|   IBIS model for TI xxx DSP
[IBIS Ver]   5.1
[Disclaimer]   Please be aware that in the absence of a written agreement
|   Texas Instruments(TI) assumes no liability for:
|   (1) The accuracy of the IBIS models provided to your company,
|   however, the IBIS model is compliant to industry standard
|   IQ Level 2a.  Refer to IBIS Quality Section below for
|   for full details.
|   (2) The proper functioning of these Models in your design
|   or for any resulting applications
|   (3) Infringement of patents, copyrights or intellectual
|   property rights resulting from your use of these
|   models.
|   TI provides IBIS Models as a service to our customers and
|   therefore reserves the right to limit distribution of the
|   Models.  The information is subject to change without notice.
[File Name]  j721s2_v0p3.ibs
[File Rev]   0.3
|   -Corrected differential pin mapping
[Date]   21Jun 2022
[Source]   Texas Instruments Incorporated
[Copyright]   Property of Texas Instruments Incorporated.
|   Unauthorized reproduction and/or distribution is strictly.
|   prohibited.
|   This product is protected under copyright law and trade
|   secret law as an unpublished work.
|   Created 2012,(C) Copyright 1999-2012,
|   Texas Instruments Incorporated., All Rights Reserved.
|   These commodities are under the U.S. Government
|   distribution license control. As such,they are not to be
|   re-exported without the prior approval of the U.S.
|   Department of Commerce.
[Notes]
   This file does not include AMI models for the following:
   1. PCIe
   2. CSI
   3. Display Port
   4. USB2
   5. USB3
   6. MPHY
   For SerDes simulations use Texas Instruments IBIS AMI models
   Some IV curves contain Non monotonic data points.
|   Revision History
|   GERNERAL COMMENT: All IBIS Quality Notes below reflect latest release
|   and version of IBIS File
|   File passes ibischk6.0 with 0 errors and 95 warnings
|   v0.1: Initial version
|   v0.2: Removed 4X models
|   v0.3: Corrected differential pin mapping
|   Component j721s2
[Component] j721s2
[Manufacturer] Texas Instruments
[Package]
|Variable   Typ   Min   Max
R_pkg   0.50566   0.040052   0.94543
L_pkg   3.105e-9   5.481e-10   5.565e-9
C_pkg   1.485e-12   4.706e-13   2.385e-12
[Package Model]   ibis_package_061021
[Pin]  Signal_name   model_name
H25	ATEST0   NC
L26	ATEST1   NC
T21	CAP_VDDS0	POWER
J20	CAP_VDDS0_MCU	POWER
G16	CAP_VDDS1_MCU	POWER
P21	CAP_VDDS2	POWER
H17	CAP_VDDS2_MCU	POWER
M22	CAP_VDDS5	POWER
AC20	CSI0_ATB_0_H	NC
AC19	CSI0_ATB_1_H	NC
AH19	CSI0_RXCLKN	NC
AH20	CSI0_RXCLKP	NC
AG18	CSI0_RXN0	NC
AF19	CSI0_RXN1	NC
AE18	CSI0_RXN2	NC
AD19	CSI0_RXN3	NC
AG19	CSI0_RXP0	NC
AF20	CSI0_RXP1	NC
AE19	CSI0_RXP2	NC
AD20	CSI0_RXP3	NC
AC18	CSI0_RXRCALIB	NC
AC23	CSI1_ATB_0_H	NC
AB22	CSI1_ATB_1_H	NC
AH22	CSI1_RXCLKN	NC
AH23	CSI1_RXCLKP	NC
AG21	CSI1_RXN0	NC
AF22	CSI1_RXN1	NC
AE21	CSI1_RXN2	NC
AD22	CSI1_RXN3	NC
AG22	CSI1_RXP0	NC
AF23	CSI1_RXP1	NC
AE22	CSI1_RXP2	NC
AD23	CSI1_RXP3	NC
AC21	CSI1_RXRCALIB	NC
T7	DDR0_ATB0	NC
N8	DDR0_ATB1	NC
P3	DDR0_CA0	DDR_SE
P5	DDR0_CA1	DDR_SE
N5	DDR0_CA2	DDR_SE
P2	DDR0_CA3	DDR_SE
P4	DDR0_CA4	DDR_SE
R3	DDR0_CA5	DDR_SE
R8	DDR0_CAL0	DDR_SE
R2	DDR0_CKE0	DDR_SE
R4	DDR0_CKE1	DDR_SE
R1	DDR0_CKN	DDR_DIFF
P1	DDR0_CKP	DDR_DIFF
V5	DDR0_CSN0_0	DDR_SE
W5	DDR0_CSN0_1	DDR_SE
T5	DDR0_CSN1_0	DDR_SE
U6	DDR0_CSN1_1	DDR_SE
H5	DDR0_DM0	DDR_SE
M3	DDR0_DM1	DDR_SE
U4	DDR0_DM2	DDR_SE
AD1	DDR0_DM3	DDR_SE
F3	DDR0_DQ0	DDR_SE
G4	DDR0_DQ1	DDR_SE
K3	DDR0_DQ10	DDR_SE
K1	DDR0_DQ11	DDR_SE
N4	DDR0_DQ12	DDR_SE
N2	DDR0_DQ13	DDR_SE
L4	DDR0_DQ14	DDR_SE
L2	DDR0_DQ15	DDR_SE
T1	DDR0_DQ16	DDR_SE
T3	DDR0_DQ17	DDR_SE
V3	DDR0_DQ18	DDR_SE
U2	DDR0_DQ19	DDR_SE
F5	DDR0_DQ2	DDR_SE
W2	DDR0_DQ20	DDR_SE
W4	DDR0_DQ21	DDR_SE
Y1	DDR0_DQ22	DDR_SE
Y3	DDR0_DQ23	DDR_SE
AB3	DDR0_DQ24	DDR_SE
AA2	DDR0_DQ25	DDR_SE
AA4	DDR0_DQ26	DDR_SE
Y5	DDR0_DQ27	DDR_SE
AC2	DDR0_DQ28	DDR_SE
AB5	DDR0_DQ29	DDR_SE
F1	DDR0_DQ3	DDR_SE
AD2	DDR0_DQ30	DDR_SE
AC4	DDR0_DQ31	DDR_SE
J4	DDR0_DQ4	DDR_SE
H3	DDR0_DQ5	DDR_SE
J2	DDR0_DQ6	DDR_SE
G2	DDR0_DQ7	DDR_SE
K5	DDR0_DQ8	DDR_SE
M5	DDR0_DQ9	DDR_SE
H1	DDR0_DQS0N	DDR_DIFF
G1	DDR0_DQS0P	DDR_DIFF
M1	DDR0_DQS1N	DDR_DIFF
L1	DDR0_DQS1P	DDR_DIFF
U1	DDR0_DQS2N	DDR_DIFF
V1	DDR0_DQS2P	DDR_DIFF
AC1	DDR0_DQS3N	DDR_DIFF
AB1	DDR0_DQS3P	DDR_DIFF
R5	DDR0_RESETN	DDR_SE
T8	DDR0_RET	DDR_SE
F13	DDR1_ATB0	NC
G11	DDR1_ATB1	NC
C10	DDR1_CA0	DDR_SE
E10	DDR1_CA1	DDR_SE
E9	DDR1_CA2	DDR_SE
B10	DDR1_CA3	DDR_SE
D10	DDR1_CA4	DDR_SE
C9	DDR1_CA5	DDR_SE
E8	DDR1_CAL0	DDR_SE
B9	DDR1_CKE0	DDR_SE
D9	DDR1_CKE1	DDR_SE
A9	DDR1_CKN	DDR_DIFF
A10	DDR1_CKP	DDR_DIFF
F9	DDR1_CSN0_0	DDR_SE
F8	DDR1_CSN0_1	DDR_SE
F11	DDR1_CSN1_0	DDR_SE
F10	DDR1_CSN1_1	DDR_SE
D16	DDR1_DM0	DDR_SE
E13	DDR1_DM1	DDR_SE
F7	DDR1_DM2	DDR_SE
B3	DDR1_DM3	DDR_SE
B18	DDR1_DQ0	DDR_SE
E17	DDR1_DQ1	DDR_SE
C13	DDR1_DQ10	DDR_SE
C11	DDR1_DQ11	DDR_SE
E11	DDR1_DQ12	DDR_SE
A11	DDR1_DQ13	DDR_SE
B12	DDR1_DQ14	DDR_SE
D12	DDR1_DQ15	DDR_SE
B7	DDR1_DQ16	DDR_SE
D7	DDR1_DQ17	DDR_SE
C8	DDR1_DQ18	DDR_SE
A8	DDR1_DQ19	DDR_SE
D18	DDR1_DQ2	DDR_SE
C6	DDR1_DQ20	DDR_SE
E6	DDR1_DQ21	DDR_SE
B5	DDR1_DQ22	DDR_SE
D5	DDR1_DQ23	DDR_SE
B1	DDR1_DQ24	DDR_SE
A4	DDR1_DQ25	DDR_SE
C4	DDR1_DQ26	DDR_SE
E4	DDR1_DQ27	DDR_SE
D1	DDR1_DQ28	DDR_SE
D3	DDR1_DQ29	DDR_SE
A17	DDR1_DQ3	DDR_SE
C2	DDR1_DQ30	DDR_SE
E2	DDR1_DQ31	DDR_SE
E15	DDR1_DQ4	DDR_SE
B16	DDR1_DQ5	DDR_SE
C15	DDR1_DQ6	DDR_SE
C17	DDR1_DQ7	DDR_SE
B14	DDR1_DQ8	DDR_SE
D14	DDR1_DQ9	DDR_SE
A15	DDR1_DQS0N	DDR_DIFF
A16	DDR1_DQS0P	DDR_DIFF
A12	DDR1_DQS1N	DDR_DIFF
A13	DDR1_DQS1P	DDR_DIFF
A7	DDR1_DQS2N	DDR_DIFF
A6	DDR1_DQS2P	DDR_DIFF
A2	DDR1_DQS3N	DDR_DIFF
A3	DDR1_DQS3P	DDR_DIFF
F12	DDR1_RESETN	DDR_SE
J10	DDR1_RET	DDR_SE
AE11	DP0_AUX_ATB_0	NC
AD12	DP0_AUX_ATB_1	NC
AG11	DP0_AUXN	NC
AF11	DP0_AUXP	NC
AC12	DSI0_ATB_0_H	NC
AC14	DSI0_ATB_1_H	NC
AH13	DSI0_TXCLKN	NC
AH14	DSI0_TXCLKP	NC
AG12	DSI0_TXN0	NC
AF13	DSI0_TXN1	NC
AE12	DSI0_TXN2	NC
AD13	DSI0_TXN3	NC
AG13	DSI0_TXP0	NC
AF14	DSI0_TXP1	NC
AE13	DSI0_TXP2	NC
AD14	DSI0_TXP3	NC
AC13	DSI0_TXRCALIB	NC
AC17	DSI1_ATB_0_H	NC
AC16	DSI1_ATB_1_H	NC
AH16	DSI1_TXCLKN	NC
AH17	DSI1_TXCLKP	NC
AG15	DSI1_TXN0	NC
AF16	DSI1_TXN1	NC
AE15	DSI1_TXN2	NC
AD16	DSI1_TXN3	NC
AG16	DSI1_TXP0	NC
AF17	DSI1_TXP1	NC
AE16	DSI1_TXP2	NC
AD17	DSI1_TXP3	NC
AC15	DSI1_TXRCALIB	NC
AB26	ECAP0_IN_APWM_OUT	LVCMOS_H
A27	EMU0	LVCMOS_V
C26	EMU1	LVCMOS_V
AD28	EXT_REFCLK1	LVCMOS_H
AG24	EXTINTN	IIC_H
V23	GPIO0_11	LVCMOS_H
T26	GPIO0_12	LVCMOS_H
AH25	I2C0_SCL	IIC_H
AE24	I2C0_SDA	IIC_H
N28	IFORCE	NC
L23	MAIN_ATEST	NC
U28	MCAN0_RX	LVCMOS_H
W28	MCAN0_TX	LVCMOS_H
R27	MCAN1_RX	LVCMOS_H
V26	MCAN1_TX	LVCMOS_H
AC24	MCAN12_RX	LVCMOS_H
W25	MCAN12_TX	LVCMOS_H
AF28	MCAN13_RX	LVCMOS_H
AE28	MCAN13_TX	LVCMOS_H
W23	MCAN14_RX	LVCMOS_H
AD25	MCAN14_TX	LVCMOS_H
AA23	MCAN15_RX	LVCMOS_H
Y24	MCAN15_TX	LVCMOS_H
AB24	MCAN16_RX	LVCMOS_H
Y28	MCAN16_TX	LVCMOS_H
Y25	MCAN2_RX	LVCMOS_H
R28	MCAN2_TX	LVCMOS_H
AB28	MCASP0_ACLKX	LVCMOS_H
U27	MCASP0_AFSX	LVCMOS_H
AC28	MCASP0_AXR0	LVCMOS_H
Y26	MCASP0_AXR1	LVCMOS_H
V25	MCASP0_AXR10	LVCMOS_H
T24	MCASP0_AXR11	LVCMOS_H
AB25	MCASP0_AXR12	LVCMOS_H
T23	MCASP0_AXR13	LVCMOS_H
U24	MCASP0_AXR14	LVCMOS_H
AC25	MCASP0_AXR15	LVCMOS_H
AB27	MCASP0_AXR2	LVCMOS_H
T27	MCASP0_AXR3	LVCMOS_H
U26	MCASP0_AXR4	LVCMOS_H
AA28	MCASP0_AXR5	LVCMOS_H
AD27	MCASP0_AXR6	LVCMOS_H
T25	MCASP0_AXR7	LVCMOS_H
W24	MCASP0_AXR8	LVCMOS_H
AA25	MCASP0_AXR9	LVCMOS_H
AA24	MCASP1_ACLKX	LVCMOS_H
V28	MCASP1_AFSX	LVCMOS_H
T28	MCASP1_AXR0	LVCMOS_H
V27	MCASP1_AXR1	LVCMOS_H
W27	MCASP1_AXR2	LVCMOS_H
AD26	MCASP1_AXR3	LVCMOS_H
U25	MCASP1_AXR4	LVCMOS_H
Y27	MCASP2_ACLKX	LVCMOS_H
AA27	MCASP2_AFSX	LVCMOS_H
AA26	MCASP2_AXR0	LVCMOS_H
AC27	MCASP2_AXR1	LVCMOS_H
L25	MCU_ADC0_AIN0	NC
K25	MCU_ADC0_AIN1	NC
M24	MCU_ADC0_AIN2	NC
L24	MCU_ADC0_AIN3	NC
L27	MCU_ADC0_AIN4	NC
K24	MCU_ADC0_AIN5	NC
M27	MCU_ADC0_AIN6	NC
M26	MCU_ADC0_AIN7	NC
P25	MCU_ADC1_AIN0	NC
R25	MCU_ADC1_AIN1	NC
P28	MCU_ADC1_AIN2	NC
P27	MCU_ADC1_AIN3	NC
N25	MCU_ADC1_AIN4	NC
P26	MCU_ADC1_AIN5	NC
N26	MCU_ADC1_AIN6	NC
N27	MCU_ADC1_AIN7	NC
G24	MCU_I2C0_SCL	IIC_V
J25	MCU_I2C0_SDA	IIC_V
E28	MCU_MCAN0_RX	LVCMOS_V
E27	MCU_MCAN0_TX	LVCMOS_V
A21	MCU_MDIO0_MDC	LVCMOS_V
A22	MCU_MDIO0_MDIO	LVCMOS_V
D19	MCU_OSPI0_CLK	LVCMOS_V
F15	MCU_OSPI0_CSN0	LVCMOS_V
G17	MCU_OSPI0_CSN1	LVCMOS_V
F14	MCU_OSPI0_CSN2	LVCMOS_V
F17	MCU_OSPI0_CSN3	LVCMOS_V
C19	MCU_OSPI0_D0	LVCMOS_V
F16	MCU_OSPI0_D1	LVCMOS_V
G15	MCU_OSPI0_D2	LVCMOS_V
F18	MCU_OSPI0_D3	LVCMOS_V
E19	MCU_OSPI0_D4	LVCMOS_V
G19	MCU_OSPI0_D5	LVCMOS_V
F19	MCU_OSPI0_D6	LVCMOS_V
F20	MCU_OSPI0_D7	LVCMOS_V
E18	MCU_OSPI0_DQS	LVCMOS_V
E20	MCU_OSPI0_LBCLKO	LVCMOS_V
A19	MCU_OSPI1_CLK	LVCMOS_V
D20	MCU_OSPI1_CSN0	LVCMOS_V
C21	MCU_OSPI1_CSN1	LVCMOS_V
D21	MCU_OSPI1_D0	LVCMOS_V
G20	MCU_OSPI1_D1	LVCMOS_V
C20	MCU_OSPI1_D2	LVCMOS_V
A20	MCU_OSPI1_D3	LVCMOS_V
B19	MCU_OSPI1_DQS	LVCMOS_V
B20	MCU_OSPI1_LBCLKO	LVCMOS_V
G23	MCU_PORZ	RESET_H
A23	MCU_RESETSTATZ	LVCMOS_V
A26	MCU_RESETZ	LVCMOS_V
B22	MCU_RGMII1_RD0	LVCMOS_V
B21	MCU_RGMII1_RD1	LVCMOS_V
C22	MCU_RGMII1_RD2	LVCMOS_V
D23	MCU_RGMII1_RD3	LVCMOS_V
E23	MCU_RGMII1_RX_CTL	LVCMOS_V
D22	MCU_RGMII1_RXC	LVCMOS_V
F23	MCU_RGMII1_TD0	LVCMOS_V
G22	MCU_RGMII1_TD1	LVCMOS_V
E21	MCU_RGMII1_TD2	LVCMOS_V
E22	MCU_RGMII1_TD3	LVCMOS_V
F22	MCU_RGMII1_TX_CTL	LVCMOS_V
F21	MCU_RGMII1_TXC	LVCMOS_V
J23	MCU_SAFETY_ERRORN	LVCMOS_V
B27	MCU_SPI0_CLK	LVCMOS_V
B26	MCU_SPI0_CS0	LVCMOS_V
D24	MCU_SPI0_D0	LVCMOS_V
B25	MCU_SPI0_D1	LVCMOS_V
AF1	MMC0_CALPAD	EMMC
AC6	MMC0_CLK	EMMC
AF2	MMC0_CMD	EMMC
AF4	MMC0_DAT0	EMMC
AD3	MMC0_DAT1	EMMC
AD4	MMC0_DAT2	EMMC
AF3	MMC0_DAT3	EMMC
AE2	MMC0_DAT4	EMMC
AG3	MMC0_DAT5	EMMC
AE1	MMC0_DAT6	EMMC
AG1	MMC0_DAT7	EMMC
AE3	MMC0_DS	EMMC
AD5	MMC0_VCTRL_TP	EMMC
P23	MMC1_CLK	SDIO_H
N24	MMC1_CMD	SDIO_H
M23	MMC1_DAT0	SDIO_H
P24	MMC1_DAT1	SDIO_H
R24	MMC1_DAT2	SDIO_H
R22	MMC1_DAT3	SDIO_H
M28	OSC1_XI	NC
L28	OSC1_XO	NC
AH10	PCIE_REFCLK1_N_OUT	NC
AH11	PCIE_REFCLK1_P_OUT	NC
G26	PMIC_POWER_EN1	LVCMOS_V
AD24	PMIC_WAKE0	LVCMOS_H
K23	PORZ	RESET_H
A24	RESET_REQZ	LVCMOS_V
AF27	RESETSTATZ	LVCMOS_H
AD11	SERDES0_ATB_0	NC
AD10	SERDES0_ATB_1	NC
AH4	SERDES0_REFCLK_N	NC
AH5	SERDES0_REFCLK_P	NC
AC10	SERDES0_REXT	NC
AF9	SERDES0_RX0_N	NC
AF10	SERDES0_RX0_P	NC
AE8	SERDES0_RX1_N	NC
AE9	SERDES0_RX1_P	NC
AF6	SERDES0_RX2_N	NC
AF7	SERDES0_RX2_P	NC
AE5	SERDES0_RX3_N	NC
AE6	SERDES0_RX3_P	NC
AH7	SERDES0_TX0_N	NC
AH8	SERDES0_TX0_P	NC
AG8	SERDES0_TX1_N	NC
AG9	SERDES0_TX1_P	NC
AG5	SERDES0_TX2_N	NC
AG6	SERDES0_TX2_P	NC
AD7	SERDES0_TX3_N	NC
AD8	SERDES0_TX3_P	NC
AF25	SOC_SAFETY_ERRORN	LVCMOS_H
AH27	SPI0_CLK	LVCMOS_H
AE27	SPI0_CS0	LVCMOS_H
AF26	SPI0_CS1	LVCMOS_H
AG26	SPI0_D0	LVCMOS_H
AH26	SPI0_D1	LVCMOS_H
A25	TCK	LVCMOS_V
AG28	TDI	LVCMOS_H
AE26	TDO	LVCMOS_H
G21	TEMP_DIODE_P	NC
AE25	TIMER_IO0	LVCMOS_H
AG25	TIMER_IO1	LVCMOS_H
AG27	TMS	LVCMOS_H
B28	TRSTN	LVCMOS_V
AG2	USB0_DM	NC
AH2	USB0_DP	NC
AC9	USB0_ID	NC
AA6	USB0_RCALIB	NC
AA8	USB0_VBUS	NC
J13	VDD_CORE	POWER
J15	VDD_CORE	POWER
M16	VDD_CORE	POWER
M19	VDD_CORE	POWER
N10	VDD_CORE	POWER
P18	VDD_CORE	POWER
R17	VDD_CORE	POWER
R19	VDD_CORE	POWER
T10	VDD_CORE	POWER
T20	VDD_CORE	POWER
U8	VDD_CORE	POWER
U15	VDD_CORE	POWER
U17	VDD_CORE	POWER
V7	VDD_CORE	POWER
V9	VDD_CORE	POWER
V14	VDD_CORE	POWER
V18	VDD_CORE	POWER
V20	VDD_CORE	POWER
W8	VDD_CORE	POWER
W10	VDD_CORE	POWER
W13	VDD_CORE	POWER
W15	VDD_CORE	POWER
W17	VDD_CORE	POWER
W19	VDD_CORE	POWER
W21	VDD_CORE	POWER
Y9	VDD_CORE	POWER
Y12	VDD_CORE	POWER
Y22	VDD_CORE	POWER
AA21	VDD_CORE	POWER
AB20	VDD_CORE	POWER
G8	VDD_CPU	POWER
H7	VDD_CPU	POWER
J8	VDD_CPU	POWER
K7	VDD_CPU	POWER
K9	VDD_CPU	POWER
K11	VDD_CPU	POWER
K13	VDD_CPU	POWER
L8	VDD_CPU	POWER
M7	VDD_CPU	POWER
M9	VDD_CPU	POWER
M14	VDD_CPU	POWER
N11	VDD_CPU	POWER
N15	VDD_CPU	POWER
P16	VDD_CPU	POWER
R13	VDD_CPU	POWER
R15	VDD_CPU	POWER
T12	VDD_CPU	POWER
T14	VDD_CPU	POWER
U11	VDD_CPU	POWER
U13	VDD_CPU	POWER
K16	VDD_MCU	POWER
K18	VDD_MCU	POWER
L15	VDD_MCU	POWER
L17	VDD_MCU	POWER
L19	VDD_MCU	POWER
J19	VDD_MCU_WAKE1	POWER
P20	VDD_WAKE0	POWER
AB17	VDDA_0P8_CSIRX0_1	POWER
AB18	VDDA_0P8_CSIRX0_1	POWER
W7	VDDA_0P8_DLL_MMC0	POWER
AB14	VDDA_0P8_DSITX	POWER
AB15	VDDA_0P8_DSITX_C	POWER
P10	VDDA_0P8_PLL_DDR0	POWER
J14	VDDA_0P8_PLL_DDR1	POWER
AA10	VDDA_0P8_SERDES_C0_1	POWER
AA11	VDDA_0P8_SERDES_C0_1	POWER
AB10	VDDA_0P8_SERDES0_1	POWER
AB11	VDDA_0P8_SERDES0_1	POWER
AB8	VDDA_0P8_USB	POWER
AA17	VDDA_1P8_CSIRX0_1	POWER
AA19	VDDA_1P8_CSIRX0_1	POWER
AA14	VDDA_1P8_DSITX	POWER
AA15	VDDA_1P8_DSITX	POWER
AA12	VDDA_1P8_SERDES0_1	POWER
AB13	VDDA_1P8_SERDES2_4	POWER
AB7	VDDA_1P8_USB	POWER
AB9	VDDA_3P3_USB	POWER
J21	VDDA_ADC0	POWER
K21	VDDA_ADC1	POWER
K22	VDDA_MCU_PLLGRP0	POWER
J17	VDDA_MCU_TEMP	POWER
L21	VDDA_OSC1	POWER
U18	VDDA_PLLGRP0	POWER
V19	VDDA_PLLGRP1	POWER
Y16	VDDA_PLLGRP10	POWER
Y18	VDDA_PLLGRP12	POWER
V12	VDDA_PLLGRP13	POWER
Y11	VDDA_PLLGRP2	POWER
N14	VDDA_PLLGRP5	POWER
R12	VDDA_PLLGRP6	POWER
R11	VDDA_PLLGRP7	POWER
K12	VDDA_PLLGRP8	POWER
T18	VDDA_PLLGRP9	POWER
L20	VDDA_POR_WKUP	POWER
U19	VDDA_TEMP0	POWER
K10	VDDA_TEMP1	POWER
T16	VDDA_TEMP2	POWER
U10	VDDA_TEMP3	POWER
Y14	VDDA_TEMP4	POWER
J22	VDDA_WKUP	POWER
N17	VDDAR_CORE	POWER
V11	VDDAR_CORE	POWER
V16	VDDAR_CORE	POWER
Y20	VDDAR_CORE	POWER
H9	VDDAR_CPU	POWER
K14	VDDAR_CPU	POWER
P11	VDDAR_CPU	POWER
P14	VDDAR_CPU	POWER
V13	VDDAR_CPU	POWER
K17	VDDAR_MCU	POWER
K19	VDDAR_MCU	POWER
A1	VDDS_DDR	POWER
A18	VDDS_DDR	POWER
G6	VDDS_DDR	POWER
G10	VDDS_DDR	POWER
G12	VDDS_DDR	POWER
G14	VDDS_DDR	POWER
H11	VDDS_DDR	POWER
H13	VDDS_DDR	POWER
H15	VDDS_DDR	POWER
J6	VDDS_DDR	POWER
L6	VDDS_DDR	POWER
N6	VDDS_DDR	POWER
N9	VDDS_DDR	POWER
P7	VDDS_DDR	POWER
P8	VDDS_DDR	POWER
R6	VDDS_DDR	POWER
U9	VDDS_DDR	POWER
AA1	VDDS_DDR	POWER
R9	VDDS_DDR_C0	POWER
J12	VDDS_DDR_C1	POWER
Y7	VDDS_MMC0	POWER
Y8	VDDS_MMC0	POWER
R21	VDDSHV0	POWER
U21	VDDSHV0	POWER
U22	VDDSHV0	POWER
H19	VDDSHV0_MCU	POWER
H20	VDDSHV0_MCU	POWER
H16	VDDSHV1_MCU	POWER
J16	VDDSHV1_MCU	POWER
M20	VDDSHV2	POWER
R20	VDDSHV2	POWER
G18	VDDSHV2_MCU	POWER
H18	VDDSHV2_MCU	POWER
M21	VDDSHV5	POWER
N22	VDDSHV5	POWER
H23	VMON1_ER_VSYS	POWER
M18	VMON2_IR_VCPU	POWER
L22	VMON3_IR_VEXT1P8	POWER
N19	VMON4_IR_VEXT1P8	POWER
N20	VMON5_IR_VEXT3P3	POWER
L18	VMON6_IR_VEXT1P8	POWER
V22	VPP_CORE	POWER
H22	VPP_MCU	POWER
K28	VSENSE	POWER
A5	VSS	GND
A14	VSS	GND
B2	VSS	GND
B4	VSS	GND
B6	VSS	GND
B8	VSS	GND
B11	VSS	GND
B13	VSS	GND
B15	VSS	GND
B17	VSS	GND
B23	VSS	GND
C1	VSS	GND
C3	VSS	GND
C5	VSS	GND
C7	VSS	GND
C12	VSS	GND
C14	VSS	GND
C16	VSS	GND
C18	VSS	GND
D2	VSS	GND
D4	VSS	GND
D6	VSS	GND
D8	VSS	GND
D11	VSS	GND
D13	VSS	GND
D15	VSS	GND
D17	VSS	GND
E1	VSS	GND
E3	VSS	GND
E5	VSS	GND
E7	VSS	GND
E12	VSS	GND
E14	VSS	GND
E16	VSS	GND
E26	VSS	GND
F2	VSS	GND
F4	VSS	GND
F6	VSS	GND
G3	VSS	GND
G5	VSS	GND
G7	VSS	GND
G9	VSS	GND
G13	VSS	GND
G28	VSS	GND
H2	VSS	GND
H4	VSS	GND
H6	VSS	GND
H8	VSS	GND
H10	VSS	GND
H12	VSS	GND
H14	VSS	GND
H21	VSS	GND
J1	VSS	GND
J3	VSS	GND
J5	VSS	GND
J7	VSS	GND
J9	VSS	GND
J11	VSS	GND
J18	VSS	GND
J24	VSS	GND
K2	VSS	GND
K4	VSS	GND
K6	VSS	GND
K8	VSS	GND
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|********************  DIFF PIN  *******************************
[Diff_pin]   inv_pin vdiff tdelay_typ   tdelay_min  tdelay_max
H1	G1	NA NA NA NA	||	ddr0_dqs0n	&	ddr0_dqs0p
M1	L1	NA NA NA NA	||	ddr0_dqs1n	&	ddr0_dqs1p
U1	V1	NA NA NA NA	||	ddr0_dqs2n	&	ddr0_dqs2p
AC1	AB1	NA NA NA NA	||	ddr0_dqs3n	&	ddr0_dqs3p
R1   P1	NA NA NA NA	||	ddr0_ckn	&	ddr0_ckp
A15	A16	NA NA NA NA	||	ddr1_dqs0n	&	ddr1_dqs0p
A12	A13	NA NA NA NA	||	ddr1_dqs1n	&	ddr1_dqs1p
A7	A6	NA NA NA NA	||	ddr1_dqs2n	&	ddr1_dqs2p
A2	A3	NA NA NA NA	||	ddr1_dqs3n	&	ddr1_dqs3p
A9	A10	NA NA NA NA	||	ddr1_ckn	&	ddr1_ckp
[Series Pin Mapping] pin_2 model_name function_table_group
| AC25	AD25	s_ILVDS18TH_PB300
| AD24	AE24	s_ILVDS18TH_PB300
| K21	L21	s_ILVDS18TH_PB300
|---------------- DDR -------------------
[Model Selector] DDR_SE
lpddr4_ocd_240p_240n  driver with 240 ohms pullup and 240 ohms pulldown strength
lpddr4_ocd_120p_120n  driver with 120 ohms pullup and 120 ohms pulldown strength
lpddr4_ocd_80p_80n  driver with 80 ohms pullup and 80 ohms pulldown strength
lpddr4_ocd_60p_60n  driver with 60 ohms pullup and 60 ohms pulldown strength
lpddr4_ocd_48p_48n  driver with 48 ohms pullup and 48 ohms pulldown strength
lpddr4_ocd_40p_40n  driver with 40 ohms pullup and 40 ohms pulldown strength
lpddr4_ocd_120pd_60p_40n  driver with 60/40 ohms pullup/pulldown 120 ohms aopd strength
lpddr4_ocd_120pd_48p_40n  driver with 48/40 ohms pullup/pulldown 120 ohms aopd strength
lpddr4_odt_240  240 ohm termination
lpddr4_odt_120  120 ohm termination
lpddr4_odt_80  80 ohm termination
lpddr4_odt_60  60 ohm termination
lpddr4_odt_48  48 ohm termination
lpddr4_odt_40  40 ohm termination
lpddr4_odt_off  open ohm termination
[Model Selector] DDR_DIFF
lpddr4_ocd_240p_240n_diff  driver with 240 ohms pullup and 240 ohms pulldown strength
lpddr4_ocd_120p_120n_diff  driver with 120 ohms pullup and 120 ohms pulldown strength
lpddr4_ocd_80p_80n_diff  driver with 80 ohms pullup and 80 ohms pulldown strength
lpddr4_ocd_60p_60n_diff  driver with 60 ohms pullup and 60 ohms pulldown strength
lpddr4_ocd_48p_48n_diff  driver with 48 ohms pullup and 48 ohms pulldown strength
lpddr4_ocd_40p_40n_diff  driver with 40 ohms pullup and 40 ohms pulldown strength
lpddr4_ocd_120pd_60p_40n_diff  driver with 60/40 ohms pullup/pulldown 120 ohms aopd strength
lpddr4_ocd_120pd_48p_40n_diff  driver with 48/40 ohms pullup/pulldown 120 ohms aopd strength
lpddr4_odt_240_diff  240 ohm termination
lpddr4_odt_120_diff  120 ohm termination
lpddr4_odt_80_diff  80 ohm termination
lpddr4_odt_60_diff  60 ohm termination
lpddr4_odt_48_diff  48 ohm termination
lpddr4_odt_40_diff  40 ohm termination
lpddr4_odt_off_diff  open ohm termination
|****************** SDIO
[Model Selector] SDIO_H
sdio1_r33_1p8_h PRWDWUWSWEWCDGSDIO_H@_R33_1p8_comment
sdio1_r33_3p3_h PRWDWUWSWEWCDGSDIO_H@_R33_3p3_comment
sdio1_r40_1p8_h PRWDWUWSWEWCDGSDIO_H@_R40_1p8_comment
sdio1_r40_3p3_h PRWDWUWSWEWCDGSDIO_H@_R40_3p3_comment
sdio1_r50_1p8_h PRWDWUWSWEWCDGSDIO_H@_R50_1p8_comment
sdio1_r50_3p3_h PRWDWUWSWEWCDGSDIO_H@_R50_3p3_comment
sdio1_r66_1p8_h PRWDWUWSWEWCDGSDIO_H@_R66_1p8_comment
sdio1_r66_3p3_h PRWDWUWSWEWCDGSDIO_H@_R66_3p3_comment
sdio1_utr33_1p8_h PRWDWUWSWEWCDGSDIO_H@_UT_R33_1p8_comment
sdio1_utr33_3p3_h PRWDWUWSWEWCDGSDIO_H@_UT_R33_3p3_comment
sdio1_utr40_1p8_h PRWDWUWSWEWCDGSDIO_H@_UT_R40_1p8_comment
sdio1_utr40_3p3_h PRWDWUWSWEWCDGSDIO_H@_UT_R40_3p3_comment
sdio1_utr50_1p8_h PRWDWUWSWEWCDGSDIO_H@_UT_R50_1p8_comment
sdio1_utr50_3p3_h PRWDWUWSWEWCDGSDIO_H@_UT_R50_3p3_comment
sdio1_utr66_1p8_h PRWDWUWSWEWCDGSDIO_H@_UT_R66_1p8_comment
sdio1_utr66_3p3_h PRWDWUWSWEWCDGSDIO_H@_UT_R66_3p3_comment
|********** LVCMOS
[Model Selector] LVCMOS_H
lvcmos1_nom_1p8_h PRWDWUWSWEWCDGLVCMOS_H@_Nom_1p8_comment
lvcmos1_nom_3p3_h PRWDWUWSWEWCDGLVCMOS_H@_Nom_3p3_comment
lvcmos1_slow_1p8_h PRWDWUWSWEWCDGLVCMOS_H@_Slow_1p8_comment
lvcmos1_slow_3p3_h PRWDWUWSWEWCDGLVCMOS_H@_Slow_3p3_comment
lvcmos1_fast_1p8_h PRWDWUWSWEWCDGLVCMOS_H@_Fast_1p8_comment
lvcmos1_fast_3p3_h PRWDWUWSWEWCDGLVCMOS_H@_Fast_3p3_comment
lvcmos1_utnom_1p8_h PRWDWUWSWEWCDGLVCMOS_H@_UT_Nom_1p8_comment
lvcmos1_utnom_3p3_h PRWDWUWSWEWCDGLVCMOS_H@_UT_Nom_3p3_comment
lvcmos1_utslow_1p8_h PRWDWUWSWEWCDGLVCMOS_H@_UT_Slow_1p8_comment
lvcmos1_utslow_3p3_h PRWDWUWSWEWCDGLVCMOS_H@_UT_Slow_3p3_comment
lvcmos1_utfast_1p8_h PRWDWUWSWEWCDGLVCMOS_H@_UT_Fast_1p8_comment
lvcmos1_utfast_3p3_h PRWDWUWSWEWCDGLVCMOS_H@_UT_Fast_3p3_comment
[Model Selector] LVCMOS_V
lvcmos0_nom_1p8_v PRWDWUWSWEWCDGLVCMOS_V@_Nom_1p8_comment
lvcmos0_nom_3p3_v PRWDWUWSWEWCDGLVCMOS_V@_Nom_3p3_comment
lvcmos0_slow_1p8_v PRWDWUWSWEWCDGLVCMOS_V@_Slow_1p8_comment
lvcmos0_slow_3p3_v PRWDWUWSWEWCDGLVCMOS_V@_Slow_3p3_comment
lvcmos0_fast_1p8_v PRWDWUWSWEWCDGLVCMOS_V@_Fast_1p8_comment
lvcmos0_fast_3p3_v PRWDWUWSWEWCDGLVCMOS_V@_Fast_3p3_comment
lvcmos0_utnom_1p8_v PRWDWUWSWEWCDGLVCMOS_V@_UT_Nom_1p8_comment
lvcmos0_utnom_3p3_v PRWDWUWSWEWCDGLVCMOS_V@_UT_Nom_3p3_comment
lvcmos0_utslow_1p8_v PRWDWUWSWEWCDGLVCMOS_V@_UT_Slow_1p8_comment
lvcmos0_utslow_3p3_v PRWDWUWSWEWCDGLVCMOS_V@_UT_Slow_3p3_comment
lvcmos0_utfast_1p8_v PRWDWUWSWEWCDGLVCMOS_V@_UT_Fast_1p8_comment
lvcmos0_utfast_3p3_v PRWDWUWSWEWCDGLVCMOS_V@_UT_Fast_3p3_comment
[Model Selector] IIC_H
Cell18_0_0_H PRBOPDDGZIIC_H@HSMODE_HSMCSE=0_0_comment 1.8V
Cell18_0_1_H PRBOPDDGZIIC_H@HSMODE_HSMCSE=0_1_comment 1.8V
Cell18_0_2_H PRBOPDDGZIIC_H@HSMODE_HSMCSE=1_0_comment 1.8V
Cell18_0_3_H PRBOPDDGZIIC_H@HSMODE_HSMCSE=1_1_comment 1.8V
Cell33_0_0_H PRBOPDDGZIIC_H@HSMODE_HSMCSE=0_0_comment
Cell33_0_1_H PRBOPDDGZIIC_H@HSMODE_HSMCSE=0_1_comment
Cell33_0_2_H PRBOPDDGZIIC_H@HSMODE_HSMCSE=1_0_comment
Cell33_0_3_H PRBOPDDGZIIC_H@HSMODE_HSMCSE=1_1_comment
[Model Selector] IIC_V
Cell18_1_0 PRBOPDDGZIIC_V@HSMODE_HSMCSE=0_0_comment  1.8V
Cell18_1_1 PRBOPDDGZIIC_V@HSMODE_HSMCSE=0_1_comment  1.8V
Cell18_1_2 PRBOPDDGZIIC_V@HSMODE_HSMCSE=1_0_comment  1.8V
Cell18_1_3 PRBOPDDGZIIC_V@HSMODE_HSMCSE=1_1_comment  1.8V
Cell33_1_0 PRBOPDDGZIIC_V@HSMODE_HSMCSE=0_0_comment
Cell33_1_1 PRBOPDDGZIIC_V@HSMODE_HSMCSE=0_1_comment
Cell33_1_2 PRBOPDDGZIIC_V@HSMODE_HSMCSE=1_0_comment
Cell33_1_3 PRBOPDDGZIIC_V@HSMODE_HSMCSE=1_1_comment
|***************** RESET ************************************************
[Model Selector] RESET_H
reset18_0_0 PDIDGZRESET_H
|   EMMC
[MODEL SELECTOR] EMMC
emmc51_io_tx33ohm   33ohm DRIVER
emmc51_io_tx40ohm   40ohm DRIVER
emmc51_io_tx50ohm   50ohm DRIVER
emmc51_io_tx66ohm   66ohm DRIVER
emmc51_io_tx100ohm  100ohm DRIVER
emmc51_io_txod   Open drain DRIVER
|******************** Package Model *************************************
[Define Package Model]   ibis_package_061021
[Manufacturer]   TI
[OEM]   TI
[Description]   472-pin Package
|[Number of Sections]   1
[Number of Pins]   472
[Pin Numbers]
|[Pin Name]  Net Number   Net Name   Net's All Pins
T21   | 1   CAP_VDDS0   T21
J20   | 2   CAP_VDDS0_MCU   J20
G16   | 3   CAP_VDDS1_MCU   G16
P21   | 4   CAP_VDDS2   P21
H17   | 5   CAP_VDDS2_MCU   H17
M22   | 6   CAP_VDDS5   M22
N17   | 7   VDDAR_CORE   N17
   |V16
   |V11
   |Y20
H9   | 8   VDDAR_CPU   H9
   |K14
   |P14
   |V13
   |P11
K17   | 9   VDDAR_MCU   K17
   |K19
AB17   | 10   VDDA_0P8_CSIRX0_1   AB17
   |AB18
W7   | 11   VDDA_0P8_DLL_MMC0   W7
AB14   | 12   VDDA_0P8_DSITX   AB14
AB15   | 13   VDDA_0P8_DSITX_C   AB15
P10   | 14   VDDA_0P8_PLL_DDR0   P10
J14   | 15   VDDA_0P8_PLL_DDR1   J14
AB10   | 16   VDDA_0P8_SERDES0_1   AB10
   |AB11
AA10   | 17   VDDA_0P8_SERDES_C0_1   AA10
   |AA11
AB8   | 18   VDDA_0P8_USB   AB8
AA17   | 19   VDDA_1P8_CSIRX0_1   AA17
   |AA19
AA14   | 20   VDDA_1P8_DSITX   AA14
   |AA15
AA12   | 21   VDDA_1P8_SERDES0_1   AA12
AB13   | 22   VDDA_1P8_SERDES2_4   AB13
AB7   | 23   VDDA_1P8_USB   AB7
AB9   | 24   VDDA_3P3_USB   AB9
J21   | 25   VDDA_ADC0   J21
K21   | 26   VDDA_ADC1   K21
K22   | 27   VDDA_MCU_PLLGRP0   K22
J17   | 28   VDDA_MCU_TEMP   J17
L21   | 29   VDDA_OSC1   L21
U18   | 30   VDDA_PLLGRP0   U18
V19   | 31   VDDA_PLLGRP1   V19
Y11   | 32   VDDA_PLLGRP2   Y11
N14   | 33   VDDA_PLLGRP5   N14
R12   | 34   VDDA_PLLGRP6   R12
R11   | 35   VDDA_PLLGRP7   R11
K12   | 36   VDDA_PLLGRP8   K12
T18   | 37   VDDA_PLLGRP9   T18
Y16   | 38   VDDA_PLLGRP10   Y16
Y18   | 39   VDDA_PLLGRP12   Y18
V12   | 40   VDDA_PLLGRP13   V12
L20   | 41   VDDA_POR_WKUP   L20
U19   | 42   VDDA_TEMP0   U19
K10   | 43   VDDA_TEMP1   K10
T16   | 44   VDDA_TEMP2   T16
U10   | 45   VDDA_TEMP3   U10
Y14   | 46   VDDA_TEMP4   Y14
J22   | 47   VDDA_WKUP   J22
R21   | 48   VDDSHV0   R21
   |U21
   |U22
H19   | 49   VDDSHV0_MCU   H19
   |H20
H16   | 50   VDDSHV1_MCU   H16
   |J16
M20   | 51   VDDSHV2   M20
   |R20
G18   | 52   VDDSHV2_MCU   G18
   |H18
M21   | 53   VDDSHV5   M21
   |N22
H15   | 54   VDDS_DDR   H15
   |G14
   |A1
   |A18
   |H13
   |G12
   |H11
   |G10
   |G6
   |J6
   |L6
   |N9
   |N6
   |P8
   |P7
   |R6
   |U9
   |AA1
R9   | 55   VDDS_DDR_C0   R9
J12   | 56   VDDS_DDR_C1   J12
Y7   | 57   VDDS_MMC0   Y7
   |Y8
M19   | 58   VDD_CORE   M19
   |U17
   |V18
   |W13
   |W19
   |W21
   |Y12
   |Y22
   |AA21
   |AB20
   |J15
   |J13
   |M16
   |P18
   |R19
   |R17
   |T20
   |U15
   |N10
   |T10
   |U8
   |V20
   |V14
   |V9
   |V7
   |W17
   |W15
   |W10
   |W8
   |Y9
K11   | 59   VDD_CPU   K11
   |K13
   |K9
   |M14
   |N11
   |R13
   |T12
   |U11
   |U13
   |N15
   |P16
   |R15
   |T14
   |H7
   |G8
   |J8
   |K7
   |L8
   |M9
   |M7
K16   | 60   VDD_MCU   K16
   |K18
   |L15
   |L17
   |L19
J19   | 61   VDD_MCU_WAKE1   J19
P20   | 62   VDD_WAKE0   P20
V22   | 63   VPP_CORE   V22
H22   | 64   VPP_MCU   H22
H25   | 65   ATEST0   H25
L26   | 66   ATEST1   L26
AC20   | 67   CSI0_ATB_0_H   AC20
AC19   | 68   CSI0_ATB_1_H   AC19
AH19   | 69   CSI0_RXCLKN   AH19
AH20   | 70   CSI0_RXCLKP   AH20
AG18   | 71   CSI0_RXN0   AG18
AF19   | 72   CSI0_RXN1   AF19
AE18   | 73   CSI0_RXN2   AE18
AD19   | 74   CSI0_RXN3   AD19
AG19   | 75   CSI0_RXP0   AG19
AF20   | 76   CSI0_RXP1   AF20
AE19   | 77   CSI0_RXP2   AE19
AD20   | 78   CSI0_RXP3   AD20
AC18   | 79   CSI0_RXRCALIB   AC18
AC23   | 80   CSI1_ATB_0_H   AC23
AB22   | 81   CSI1_ATB_1_H   AB22
AH22   | 82   CSI1_RXCLKN   AH22
AH23   | 83   CSI1_RXCLKP   AH23
AG21   | 84   CSI1_RXN0   AG21
AF22   | 85   CSI1_RXN1   AF22
AE21   | 86   CSI1_RXN2   AE21
AD22   | 87   CSI1_RXN3   AD22
AG22   | 88   CSI1_RXP0   AG22
AF23   | 89   CSI1_RXP1   AF23
AE22   | 90   CSI1_RXP2   AE22
AD23   | 91   CSI1_RXP3   AD23
AC21   | 92   CSI1_RXRCALIB   AC21
T7   | 93   DDR0_ATB0   T7
N8   | 94   DDR0_ATB1   N8
P3   | 95   DDR0_CA0   P3
P5   | 96   DDR0_CA1   P5
N5   | 97   DDR0_CA2   N5
P2   | 98   DDR0_CA3   P2
P4   | 99   DDR0_CA4   P4
R3   | 100   DDR0_CA5   R3
R8   | 101   DDR0_CAL0   R8
R2   | 102   DDR0_CKE0   R2
R4   | 103   DDR0_CKE1   R4
R1   | 104   DDR0_CKN   R1
P1   | 105   DDR0_CKP   P1
V5   | 106   DDR0_CSN0_0   V5
W5   | 107   DDR0_CSN0_1   W5
T5   | 108   DDR0_CSN1_0   T5
U6   | 109   DDR0_CSN1_1   U6
H5   | 110   DDR0_DM0   H5
M3   | 111   DDR0_DM1   M3
U4   | 112   DDR0_DM2   U4
AD1   | 113   DDR0_DM3   AD1
F3   | 114   DDR0_DQ0   F3
G4   | 115   DDR0_DQ1   G4
F5   | 116   DDR0_DQ2   F5
F1   | 117   DDR0_DQ3   F1
J4   | 118   DDR0_DQ4   J4
H3   | 119   DDR0_DQ5   H3
J2   | 120   DDR0_DQ6   J2
G2   | 121   DDR0_DQ7   G2
K5   | 122   DDR0_DQ8   K5
M5   | 123   DDR0_DQ9   M5
K3   | 124   DDR0_DQ10   K3
K1   | 125   DDR0_DQ11   K1
N4   | 126   DDR0_DQ12   N4
N2   | 127   DDR0_DQ13   N2
L4   | 128   DDR0_DQ14   L4
L2   | 129   DDR0_DQ15   L2
T1   | 130   DDR0_DQ16   T1
T3   | 131   DDR0_DQ17   T3
V3   | 132   DDR0_DQ18   V3
U2   | 133   DDR0_DQ19   U2
W2   | 134   DDR0_DQ20   W2
W4   | 135   DDR0_DQ21   W4
Y1   | 136   DDR0_DQ22   Y1
Y3   | 137   DDR0_DQ23   Y3
AB3   | 138   DDR0_DQ24   AB3
AA2   | 139   DDR0_DQ25   AA2
AA4   | 140   DDR0_DQ26   AA4
Y5   | 141   DDR0_DQ27   Y5
AC2   | 142   DDR0_DQ28   AC2
AB5   | 143   DDR0_DQ29   AB5
AD2   | 144   DDR0_DQ30   AD2
AC4   | 145   DDR0_DQ31   AC4
H1   | 146   DDR0_DQS0N   H1
G1   | 147   DDR0_DQS0P   G1
M1   | 148   DDR0_DQS1N   M1
L1   | 149   DDR0_DQS1P   L1
U1   | 150   DDR0_DQS2N   U1
V1   | 151   DDR0_DQS2P   V1
AC1   | 152   DDR0_DQS3N   AC1
AB1   | 153   DDR0_DQS3P   AB1
R5   | 154   DDR0_RESETN   R5
T8   | 155   DDR0_RET   T8
F13   | 156   DDR1_ATB0   F13
G11   | 157   DDR1_ATB1   G11
C10   | 158   DDR1_CA0   C10
E10   | 159   DDR1_CA1   E10
E9   | 160   DDR1_CA2   E9
B10   | 161   DDR1_CA3   B10
D10   | 162   DDR1_CA4   D10
C9   | 163   DDR1_CA5   C9
E8   | 164   DDR1_CAL0   E8
B9   | 165   DDR1_CKE0   B9
D9   | 166   DDR1_CKE1   D9
A9   | 167   DDR1_CKN   A9
A10   | 168   DDR1_CKP   A10
F9   | 169   DDR1_CSN0_0   F9
F8   | 170   DDR1_CSN0_1   F8
F11   | 171   DDR1_CSN1_0   F11
F10   | 172   DDR1_CSN1_1   F10
D16   | 173   DDR1_DM0   D16
E13   | 174   DDR1_DM1   E13
F7   | 175   DDR1_DM2   F7
B3   | 176   DDR1_DM3   B3
B18   | 177   DDR1_DQ0   B18
E17   | 178   DDR1_DQ1   E17
D18   | 179   DDR1_DQ2   D18
A17   | 180   DDR1_DQ3   A17
E15   | 181   DDR1_DQ4   E15
B16   | 182   DDR1_DQ5   B16
C15   | 183   DDR1_DQ6   C15
C17   | 184   DDR1_DQ7   C17
B14   | 185   DDR1_DQ8   B14
D14   | 186   DDR1_DQ9   D14
C13   | 187   DDR1_DQ10   C13
C11   | 188   DDR1_DQ11   C11
E11   | 189   DDR1_DQ12   E11
A11   | 190   DDR1_DQ13   A11
B12   | 191   DDR1_DQ14   B12
D12   | 192   DDR1_DQ15   D12
B7   | 193   DDR1_DQ16   B7
D7   | 194   DDR1_DQ17   D7
C8   | 195   DDR1_DQ18   C8
A8   | 196   DDR1_DQ19   A8
C6   | 197   DDR1_DQ20   C6
E6   | 198   DDR1_DQ21   E6
B5   | 199   DDR1_DQ22   B5
D5   | 200   DDR1_DQ23   D5
B1   | 201   DDR1_DQ24   B1
A4   | 202   DDR1_DQ25   A4
C4   | 203   DDR1_DQ26   C4
E4   | 204   DDR1_DQ27   E4
D1   | 205   DDR1_DQ28   D1
D3   | 206   DDR1_DQ29   D3
C2   | 207   DDR1_DQ30   C2
E2   | 208   DDR1_DQ31   E2
A15   | 209   DDR1_DQS0N   A15
A16   | 210   DDR1_DQS0P   A16
A12   | 211   DDR1_DQS1N   A12
A13   | 212   DDR1_DQS1P   A13
A7   | 213   DDR1_DQS2N   A7
A6   | 214   DDR1_DQS2P   A6
A2   | 215   DDR1_DQS3N   A2
A3   | 216   DDR1_DQS3P   A3
F12   | 217   DDR1_RESETN   F12
J10   | 218   DDR1_RET   J10
AG11   | 219   DP0_AUXN   AG11
AF11   | 220   DP0_AUXP   AF11
AE11   | 221   DP0_AUX_ATB_0   AE11
AD12   | 222   DP0_AUX_ATB_1   AD12
AC12   | 223   DSI0_ATB_0_H   AC12
AC14   | 224   DSI0_ATB_1_H   AC14
AH13   | 225   DSI0_TXCLKN   AH13
AH14   | 226   DSI0_TXCLKP   AH14
AG12   | 227   DSI0_TXN0   AG12
AF13   | 228   DSI0_TXN1   AF13
AE12   | 229   DSI0_TXN2   AE12
AD13   | 230   DSI0_TXN3   AD13
AG13   | 231   DSI0_TXP0   AG13
AF14   | 232   DSI0_TXP1   AF14
AE13   | 233   DSI0_TXP2   AE13
AD14   | 234   DSI0_TXP3   AD14
AC13   | 235   DSI0_TXRCALIB   AC13
AC17   | 236   DSI1_ATB_0_H   AC17
AC16   | 237   DSI1_ATB_1_H   AC16
AH16   | 238   DSI1_TXCLKN   AH16
AH17   | 239   DSI1_TXCLKP   AH17
AG15   | 240   DSI1_TXN0   AG15
AF16   | 241   DSI1_TXN1   AF16
AE15   | 242   DSI1_TXN2   AE15
AD16   | 243   DSI1_TXN3   AD16
AG16   | 244   DSI1_TXP0   AG16
AF17   | 245   DSI1_TXP1   AF17
AE16   | 246   DSI1_TXP2   AE16
AD17   | 247   DSI1_TXP3   AD17
AC15   | 248   DSI1_TXRCALIB   AC15
AB26   | 249   ECAP0_IN_APWM_OUT   AB26
A27   | 250   EMU0   A27
C26   | 251   EMU1   C26
AG24   | 252   EXTINTN   AG24
AD28   | 253   EXT_REFCLK1   AD28
V23   | 254   GPIO0_11   V23
T26   | 255   GPIO0_12   T26
AH25   | 256   I2C0_SCL   AH25
AE24   | 257   I2C0_SDA   AE24
N28   | 258   IFORCE   N28
L23   | 259   MAIN_ATEST   L23
U28   | 260   MCAN0_RX   U28
W28   | 261   MCAN0_TX   W28
R27   | 262   MCAN1_RX   R27
V26   | 263   MCAN1_TX   V26
Y25   | 264   MCAN2_RX   Y25
R28   | 265   MCAN2_TX   R28
AC24   | 266   MCAN12_RX   AC24
W25   | 267   MCAN12_TX   W25
AF28   | 268   MCAN13_RX   AF28
AE28   | 269   MCAN13_TX   AE28
W23   | 270   MCAN14_RX   W23
AD25   | 271   MCAN14_TX   AD25
AA23   | 272   MCAN15_RX   AA23
Y24   | 273   MCAN15_TX   Y24
AB24   | 274   MCAN16_RX   AB24
Y28   | 275   MCAN16_TX   Y28
AB28   | 276   MCASP0_ACLKX   AB28
U27   | 277   MCASP0_AFSX   U27
AC28   | 278   MCASP0_AXR0   AC28
Y26   | 279   MCASP0_AXR1   Y26
AB27   | 280   MCASP0_AXR2   AB27
T27   | 281   MCASP0_AXR3   T27
U26   | 282   MCASP0_AXR4   U26
AA28   | 283   MCASP0_AXR5   AA28
AD27   | 284   MCASP0_AXR6   AD27
T25   | 285   MCASP0_AXR7   T25
W24   | 286   MCASP0_AXR8   W24
AA25   | 287   MCASP0_AXR9   AA25
V25   | 288   MCASP0_AXR10   V25
T24   | 289   MCASP0_AXR11   T24
AB25   | 290   MCASP0_AXR12   AB25
T23   | 291   MCASP0_AXR13   T23
U24   | 292   MCASP0_AXR14   U24
AC25   | 293   MCASP0_AXR15   AC25
AA24   | 294   MCASP1_ACLKX   AA24
V28   | 295   MCASP1_AFSX   V28
T28   | 296   MCASP1_AXR0   T28
V27   | 297   MCASP1_AXR1   V27
W27   | 298   MCASP1_AXR2   W27
AD26   | 299   MCASP1_AXR3   AD26
U25   | 300   MCASP1_AXR4   U25
Y27   | 301   MCASP2_ACLKX   Y27
AA27   | 302   MCASP2_AFSX   AA27
AA26   | 303   MCASP2_AXR0   AA26
AC27   | 304   MCASP2_AXR1   AC27
L25   | 305   MCU_ADC0_AIN0   L25
K25   | 306   MCU_ADC0_AIN1   K25
M24   | 307   MCU_ADC0_AIN2   M24
L24   | 308   MCU_ADC0_AIN3   L24
L27   | 309   MCU_ADC0_AIN4   L27
K24   | 310   MCU_ADC0_AIN5   K24
M27   | 311   MCU_ADC0_AIN6   M27
M26   | 312   MCU_ADC0_AIN7   M26
P25   | 313   MCU_ADC1_AIN0   P25
R25   | 314   MCU_ADC1_AIN1   R25
P28   | 315   MCU_ADC1_AIN2   P28
P27   | 316   MCU_ADC1_AIN3   P27
N25   | 317   MCU_ADC1_AIN4   N25
P26   | 318   MCU_ADC1_AIN5   P26
N26   | 319   MCU_ADC1_AIN6   N26
N27   | 320   MCU_ADC1_AIN7   N27
G24   | 321   MCU_I2C0_SCL   G24
J25   | 322   MCU_I2C0_SDA   J25
E28   | 323   MCU_MCAN0_RX   E28
E27   | 324   MCU_MCAN0_TX   E27
A21   | 325   MCU_MDIO0_MDC   A21
A22   | 326   MCU_MDIO0_MDIO   A22
D19   | 327   MCU_OSPI0_CLK   D19
F15   | 328   MCU_OSPI0_CSN0   F15
G17   | 329   MCU_OSPI0_CSN1   G17
F14   | 330   MCU_OSPI0_CSN2   F14
F17   | 331   MCU_OSPI0_CSN3   F17
C19   | 332   MCU_OSPI0_D0   C19
F16   | 333   MCU_OSPI0_D1   F16
G15   | 334   MCU_OSPI0_D2   G15
F18   | 335   MCU_OSPI0_D3   F18
E19   | 336   MCU_OSPI0_D4   E19
G19   | 337   MCU_OSPI0_D5   G19
F19   | 338   MCU_OSPI0_D6   F19
F20   | 339   MCU_OSPI0_D7   F20
E18   | 340   MCU_OSPI0_DQS   E18
E20   | 341   MCU_OSPI0_LBCLKO   E20
A19   | 342   MCU_OSPI1_CLK   A19
D20   | 343   MCU_OSPI1_CSN0   D20
C21   | 344   MCU_OSPI1_CSN1   C21
D21   | 345   MCU_OSPI1_D0   D21
G20   | 346   MCU_OSPI1_D1   G20
C20   | 347   MCU_OSPI1_D2   C20
A20   | 348   MCU_OSPI1_D3   A20
B19   | 349   MCU_OSPI1_DQS   B19
B20   | 350   MCU_OSPI1_LBCLKO   B20
G23   | 351   MCU_PORZ   G23
A23   | 352   MCU_RESETSTATZ   A23
A26   | 353   MCU_RESETZ   A26
B22   | 354   MCU_RGMII1_RD0   B22
B21   | 355   MCU_RGMII1_RD1   B21
C22   | 356   MCU_RGMII1_RD2   C22
D23   | 357   MCU_RGMII1_RD3   D23
D22   | 358   MCU_RGMII1_RXC   D22
E23   | 359   MCU_RGMII1_RX_CTL   E23
F23   | 360   MCU_RGMII1_TD0   F23
G22   | 361   MCU_RGMII1_TD1   G22
E21   | 362   MCU_RGMII1_TD2   E21
E22   | 363   MCU_RGMII1_TD3   E22
F21   | 364   MCU_RGMII1_TXC   F21
F22   | 365   MCU_RGMII1_TX_CTL   F22
J23   | 366   MCU_SAFETY_ERRORN   J23
B27   | 367   MCU_SPI0_CLK   B27
B26   | 368   MCU_SPI0_CS0   B26
D24   | 369   MCU_SPI0_D0   D24
B25   | 370   MCU_SPI0_D1   B25
AF1   | 371   MMC0_CALPAD   AF1
AC6   | 372   MMC0_CLK   AC6
AF2   | 373   MMC0_CMD   AF2
AF4   | 374   MMC0_DAT0   AF4
AD3   | 375   MMC0_DAT1   AD3
AD4   | 376   MMC0_DAT2   AD4
AF3   | 377   MMC0_DAT3   AF3
AE2   | 378   MMC0_DAT4   AE2
AG3   | 379   MMC0_DAT5   AG3
AE1   | 380   MMC0_DAT6   AE1
AG1   | 381   MMC0_DAT7   AG1
AE3   | 382   MMC0_DS   AE3
AD5   | 383   MMC0_VCTRL_TP   AD5
P23   | 384   MMC1_CLK   P23
N24   | 385   MMC1_CMD   N24
M23   | 386   MMC1_DAT0   M23
P24   | 387   MMC1_DAT1   P24
R24   | 388   MMC1_DAT2   R24
R22   | 389   MMC1_DAT3   R22
M28   | 390   OSC1_XI   M28
L28   | 391   OSC1_XO   L28
AH10   | 392   PCIE_REFCLK1_N_OUT   AH10
AH11   | 393   PCIE_REFCLK1_P_OUT   AH11
G26   | 394   PMIC_POWER_EN1   G26
AD24   | 395   PMIC_WAKE0   AD24
K23   | 396   PORZ   K23
AF27   | 397   RESETSTATZ   AF27
A24   | 398   RESET_REQZ   A24
AD11   | 399   SERDES0_ATB_0   AD11
AD10   | 400   SERDES0_ATB_1   AD10
AH4   | 401   SERDES0_REFCLK_N   AH4
AH5   | 402   SERDES0_REFCLK_P   AH5
AC10   | 403   SERDES0_REXT   AC10
AF9   | 404   SERDES0_RX0_N   AF9
AF10   | 405   SERDES0_RX0_P   AF10
AE8   | 406   SERDES0_RX1_N   AE8
AE9   | 407   SERDES0_RX1_P   AE9
AF6   | 408   SERDES0_RX2_N   AF6
AF7   | 409   SERDES0_RX2_P   AF7
AE5   | 410   SERDES0_RX3_N   AE5
AE6   | 411   SERDES0_RX3_P   AE6
AH7   | 412   SERDES0_TX0_N   AH7
AH8   | 413   SERDES0_TX0_P   AH8
AG8   | 414   SERDES0_TX1_N   AG8
AG9   | 415   SERDES0_TX1_P   AG9
AG5   | 416   SERDES0_TX2_N   AG5
AG6   | 417   SERDES0_TX2_P   AG6
AD7   | 418   SERDES0_TX3_N   AD7
AD8   | 419   SERDES0_TX3_P   AD8
AF25   | 420   SOC_SAFETY_ERRORN   AF25
AH27   | 421   SPI0_CLK   AH27
AE27   | 422   SPI0_CS0   AE27
AF26   | 423   SPI0_CS1   AF26
AG26   | 424   SPI0_D0   AG26
AH26   | 425   SPI0_D1   AH26
A25   | 426   TCK   A25
AG28   | 427   TDI   AG28
AE26   | 428   TDO   AE26
G21   | 429   TEMP_DIODE_P   G21
AE25   | 430   TIMER_IO0   AE25
AG25   | 431   TIMER_IO1   AG25
AG27   | 432   TMS   AG27
B28   | 433   TRSTN   B28
AG2   | 434   USB0_DM   AG2
AH2   | 435   USB0_DP   AH2
AC9   | 436   USB0_ID   AC9
AA6   | 437   USB0_RCALIB   AA6
AA8   | 438   USB0_VBUS   AA8
H23   | 439   VMON1_ER_VSYS   H23
M18   | 440   VMON2_IR_VCPU   M18
L22   | 441   VMON3_IR_VEXT1P8   L22
N19   | 442   VMON4_IR_VEXT1P8   N19
N20   | 443   VMON5_IR_VEXT3P3   N20
L18   | 444   VMON6_IR_VEXT1P8   L18
K28   | 445   VSENSE   K28
D26   | 446   WKUP_GPIO0_0   D26
E24   | 447   WKUP_GPIO0_1   E24
C28   | 448   WKUP_GPIO0_2   C28
C27   | 449   WKUP_GPIO0_3   C27
C23   | 450   WKUP_GPIO0_4   C23
F26   | 451   WKUP_GPIO0_5   F26
E25   | 452   WKUP_GPIO0_6   E25
F28   | 453   WKUP_GPIO0_7   F28
F24   | 454   WKUP_GPIO0_8   F24
H26   | 455   WKUP_GPIO0_9   H26
F27   | 456   WKUP_GPIO0_10   F27
F25   | 457   WKUP_GPIO0_11   F25
C25   | 458   WKUP_GPIO0_12   C25
C24   | 459   WKUP_GPIO0_13   C24
B24   | 460   WKUP_GPIO0_14   B24
D25   | 461   WKUP_GPIO0_15   D25
K26   | 462   WKUP_GPIO0_49   K26
G27   | 463   WKUP_GPIO0_56   G27
J26   | 464   WKUP_GPIO0_57   J26
G25   | 465   WKUP_GPIO0_66   G25
J27   | 466   WKUP_GPIO0_67   J27
H24   | 467   WKUP_I2C0_SCL   H24
H27   | 468   WKUP_I2C0_SDA   H27
H28   | 469   WKUP_OSC0_XI   H28
J28   | 470   WKUP_OSC0_XO   J28
D28   | 471   WKUP_UART0_RXD   D28
D27   | 472   WKUP_UART0_TXD   D27
[Model Data]
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[End Model Data]
[End Package Model]
| Models and submodels in the file (93): lvcmos1_nom_1p8_h (I/O), lvcmos0_nom_1p8_v (I/O), lvcmos1_nom_3p3_h (I/O), lvcmos0_nom_3p3_v (I/O), lvcmos1_slow_1p8_h (I/O), lvcmos0_slow_1p8_v (I/O), lvcmos1_slow_3p3_h (I/O), lvcmos0_slow_3p3_v (I/O), lvcmos1_fast_1p8_h (I/O), lvcmos0_fast_1p8_v (I/O), lvcmos1_fast_3p3_h (I/O), lvcmos0_fast_3p3_v (I/O), lvcmos1_utnom_1p8_h (I/O), lvcmos0_utnom_1p8_v (I/O), lvcmos1_utnom_3p3_h (I/O), lvcmos0_utnom_3p3_v (I/O), lvcmos1_utslow_1p8_h (I/O), lvcmos0_utslow_1p8_v (I/O), lvcmos1_utslow_3p3_h (I/O), lvcmos0_utslow_3p3_v (I/O), lvcmos1_utfast_1p8_h (I/O), lvcmos0_utfast_1p8_v (I/O), lvcmos1_utfast_3p3_h (I/O), lvcmos0_utfast_3p3_v (I/O), sdio1_r33_1p8_h (I/O), sdio1_r33_3p3_h (I/O), sdio1_r40_1p8_h (I/O), sdio1_r40_3p3_h (I/O), sdio1_r50_1p8_h (I/O), sdio1_r50_3p3_h (I/O), sdio1_r66_1p8_h (I/O), sdio1_r66_3p3_h (I/O), sdio1_utr33_1p8_h (I/O), sdio1_utr33_3p3_h (I/O), sdio1_utr40_1p8_h (I/O), sdio1_utr40_3p3_h (I/O), sdio1_utr50_1p8_h (I/O), sdio1_utr50_3p3_h (I/O), sdio1_utr66_1p8_h (I/O), sdio1_utr66_3p3_h (I/O), lpddr4_odt_120 (Input), lpddr4_odt_120_diff (Input), lpddr4_ocd_120p_120n (I/O), lpddr4_ocd_240p_240n (I/O), lpddr4_odt_240 (Input), lpddr4_ocd_40p_40n (I/O), lpddr4_odt_40 (Input), lpddr4_ocd_48p_48n (I/O), lpddr4_odt_48 (Input), lpddr4_ocd_60p_60n (I/O), lpddr4_odt_60 (Input), lpddr4_ocd_80p_80n (I/O), lpddr4_odt_80 (Input), lpddr4_odt_off (Input), lpddr4_ocd_120pd_60p_40n (I/O), lpddr4_ocd_120p_120n_diff (I/O), lpddr4_ocd_240p_240n_diff (I/O), lpddr4_odt_240_diff (Input), lpddr4_ocd_40p_40n_diff (I/O), lpddr4_odt_40_diff (Input), lpddr4_ocd_48p_48n_diff (I/O), lpddr4_odt_48_diff (Input), lpddr4_ocd_60p_60n_diff (I/O), lpddr4_odt_60_diff (Input), lpddr4_ocd_80p_80n_diff (I/O), lpddr4_ocd_120pd_60p_40n_diff (I/O), lpddr4_odt_80_diff (Input), lpddr4_odt_off_diff (Input), lpddr4_ocd_120pd_48p_40n (I/O), lpddr4_ocd_120pd_48p_40n_diff (I/O), emmc51_io_tx33ohm (I/O), emmc51_io_tx40ohm (I/O), emmc51_io_tx50ohm (I/O), emmc51_io_tx66ohm (I/O), emmc51_io_tx100ohm (I/O), emmc51_io_txod (I/O_open_drain), Cell18_0_0_H (I/O_open_drain), Cell18_0_1_H (I/O_open_drain), Cell18_0_2_H (I/O_open_drain), Cell18_0_3_H (I/O_open_drain)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
